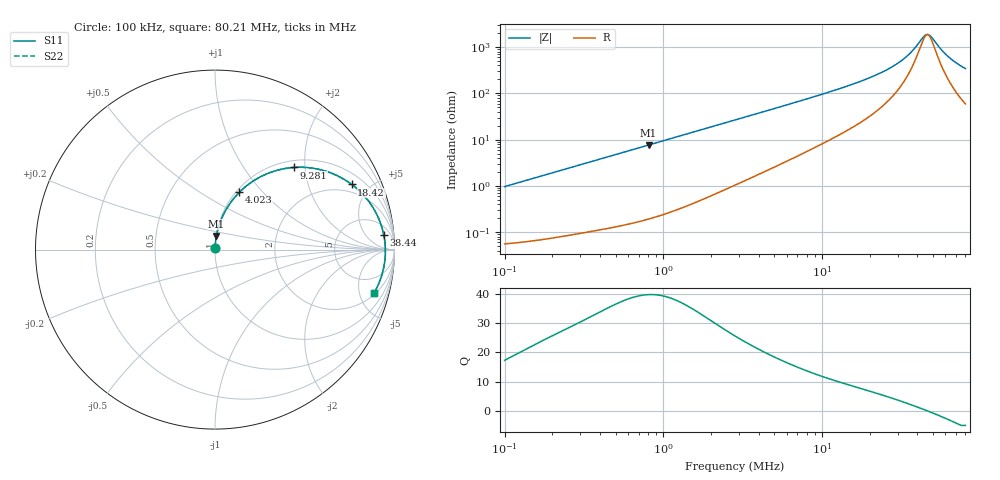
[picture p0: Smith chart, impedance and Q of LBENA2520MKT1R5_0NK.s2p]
! LBENA2520MKT1R5_0NK  S-PARAMETER MODEL  ( General Type )
! Model Generated by TAIYO YUDEN Corporation (http://www.ty-top.com)
! Version 1.0
! TAIYO YUDEN Control No. 220120
! Copyright(c) 2022 TAIYO YUDEN CO.,LTD. All Rights Reserved.
! Product Description (link to TY-COMPAS)
! https://ds.yuden.co.jp/TYCOMPAS/or/detail?pn=LBENA2520MKT1R5M0NK&u=M
! Products Name : Inductors
! Characteristics :
!  Inductance : 1.5 uH , SRF(min) : -Hz , DC Resistance(max) : 0.057 Ohm
!  Rated Current : Saturation :3300 mA , Temp Rise : 2800 mA
!  Case Size : 2.5 x 2.0 / 0.098 x 0.079 [mm/inch] , Thickness : 1.2 / 0.047 [mm/inch]
!  (Conditions: Temperature = 25 degC , DC Bias Current/Voltage = 0A / 0V)
! External Node Assignments :
!  1  o---GGG---o  2
! GND o---------o GND
! Frequency Range : 0.1MHz  -  80.209071MHz  [ 402 STEP ]
# MHz S RI R 50
! Freq[MHz].  S11 Real  S11 Imag  S21 Real  S21 Imag  S12 Real  S12 Imag  S22 Real  S22 Imag
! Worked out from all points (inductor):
!   401 points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, 100 kHz to 80.21 MHz, reference 50 ohm
!   read as one part in series: L = 1.53 uH near 103.4 kHz
!   highest Q = 39.7 at 808.3 kHz (marker M1), where L = 1.51 uH
!   self-resonance near 46.12 MHz
!   S11 on the Smith chart (normalised r, x): 100 kHz: 1.00, +0.02; 4.023 MHz: 1.04, +0.75; 9.281 MHz: 1.14, +1.76; 18.42 MHz: 1.53, +3.85; 38.44 MHz: 11, +16; 80.21 MHz: 2.18, -6.74
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0.1  0.000651 0.00964  0.9993 -0.00964  0.9993 -0.00964  0.000651 0.00964
0.306519  0.00181 0.0292  0.9982 -0.0292  0.9982 -0.0292  0.00181 0.0292
0.808295  0.0077 0.0757  0.9923 -0.0757  0.9923 -0.0757  0.0077 0.0757
0.939539  0.01 0.0877  0.99 -0.0877  0.99 -0.0877  0.01 0.0877
1.658723  0.0281 0.1511  0.9719 -0.1511  0.9719 -0.1511  0.0281 0.1511
2.832121  0.0742 0.2433  0.9258 -0.2433  0.9258 -0.2433  0.0742 0.2433
4.02331  0.1357 0.3194  0.8643 -0.3194  0.8643 -0.3194  0.1357 0.3194
5.811868  0.2415 0.3993  0.7585 -0.3993  0.7585 -0.3993  0.2415 0.3993
8.680988  0.4094 0.4547  0.5906 -0.4547  0.5906 -0.4547  0.4094 0.4547
9.281356  0.4414 0.4579  0.5586 -0.4579  0.5586 -0.4579  0.4414 0.4579
12.9665  0.6056 0.4403  0.3944 -0.4403  0.3944 -0.4403  0.6056 0.4403
18.4202  0.7618 0.3631  0.2382 -0.3631  0.2382 -0.3631  0.7618 0.3631
26.60888  0.8799 0.2345  0.1201 -0.2345  0.1201 -0.2345  0.8799 0.2345
32.52021  0.9203 0.1523  0.0797 -0.1523  0.0797 -0.1523  0.9203 0.1523
38.43783  0.9406 0.0804  0.0594 -0.0804  0.0594 -0.0804  0.9406 0.0804
43.93831  0.9483 0.0216  0.0517 -0.0216  0.0517 -0.0216  0.9483 0.0216
46.97704  0.9493 -0.00813  0.0507 0.00813  0.0507 0.00813  0.9493 -0.00813
49.39321  0.9488 -0.0305  0.0512 0.0305  0.0512 0.0305  0.9488 -0.0305
56.46141  0.942 -0.09  0.058 0.09  0.058 0.09  0.942 -0.09
62.41876  0.9317 -0.1345  0.0683 0.1345  0.0683 0.1345  0.9317 -0.1345
71.35092  0.9108 -0.193  0.0892 0.193  0.0892 0.193  0.9108 -0.193
80.20907  0.8855 -0.2428  0.1145 0.2428  0.1145 0.2428  0.8855 -0.2428
